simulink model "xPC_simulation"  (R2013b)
settings: Solver=FixedStepDiscrete  SolverMode=MultiTasking  StartTime=0.0  StopTime=inf  FixedStep=1/Param.Fs  RelTol=1e-3
InitFcn:
  | clear all; clc; close all;
  | Param  = Config_parameter();
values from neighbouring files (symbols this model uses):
  FFTLen = 2^(ceil(log(nFrmLen)/log(2)))    [DFT_FilterBank_Analysis_func.m]    (also in DFT_FilterBank_Synthesis_func.m; main_run3.m)
  nHopSize = size(in_frame_seg,1)    [DFT_FilterBank_Analysis_func.m]    (also in DFT_FilterBank_Synthesis_func.m = size(ref_out,1); main_run3.m = 16)
  nNumChs = size(ref_out,1)    [DFT_FilterBank_Analysis_func.m]    (also in DFT_FilterBank_Synthesis_func.m = size(in_frame,2); main_run3.m = 32; OLA_func.m = size(in_frame,2); PDbranchingsmooth_sm.m = size(x,1))
undefined symbols (not defined in the file or in its folder): a_dd, AFC_switch, DownSample_factor, DownSamplingFactor, eta, Freq_shift, Fs, Input, mu, prototype_win, Range, VarAmpSwitch, VarAttackTime, VarCompressRatio, VarCompressTh, VarFs, VarKneeWidth, VarLimiterCompressRatio, VarLimiterTh, VarMaxSPL, VarMicNoiseCompressRatio, VarMicNoiseTh, VarRefGaindB, VarRefSPL, VarReleaseTime, VarSwitch, VarThdB, Wiener_switch
libraries: xpcgeneralstandardslib x2, dspadpt3 x1, dspbuff3 x1, xpclib x1

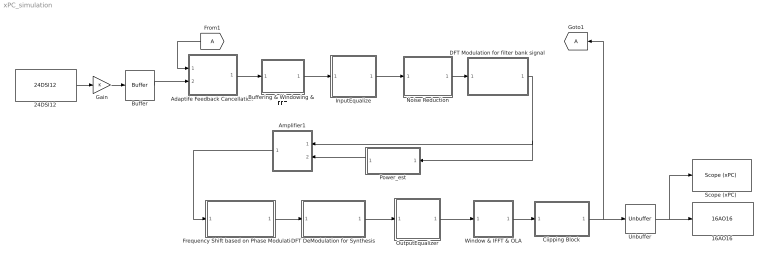
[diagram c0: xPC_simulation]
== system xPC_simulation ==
  "16AO16 " : xpcgeneralstandardslib/Audio/16AO16   channel=[1]  range=+-10.0  gsense=off  clksrc=External: slave to 24DSI12  framesize=1  samplerate=Param.Fs  sampletime=-1  autocal=on  extsync=LVDS  slot=-1
  24DSI12 : xpcgeneralstandardslib/Audio/24DSI12  channel=[1]  range=+-10.0  framesize=1  samplerate=Param.Fs  sampletime=-1  convert="+-Input Range (+-10  +-5 or +-2.5)"  filter=Low Frequency  mode=Hardware clock/Initiator  autocal=on  extsync=LVDS  slot=-1
  Adaptife Feedback Cancellation : Subsystem
  Amplifier1 : Subsystem
  Buffer : Buffer  N=Param.IO_FrameSize  TreatMby1Signals=One channel
  Buffering & Windowing &  FFT : Subsystem
  Ciipping Block : Subsystem
  DFT DeModulation for Synthesis : Subsystem
  DFT Modulation for filter bank signal : Subsystem
  Frequency Shift based on Phase Modulation : Subsystem
  From1 : From
  Gain : Gain
  Goto1 : Goto
  InputEqualize : MATLAB Function  TreatAsAtomicUnit=on
  Noise Reduction : Subsystem
  OutputEqualizer : MATLAB Function  TreatAsAtomicUnit=on
  Power_est : Subsystem
  "Scope (xPC) " : xpclib/Misc./Scope (xPC)   scopeno=1  scopetype=Target  autostart=on  viewmode=Graphical redraw  formatstr='%15.6f'  grid=on  ylimits=[0,0]  nosamples=250  noprepostsamples=0  interleave=1  triggermode=FreeRun  triggersignal=1  trigsignalfromport=off  triggerlevel=0.0  triggerslope=Either  triggerscope=1  triggersample=0  filename=data.dat  mode=Lazy  writesize=512  autorestart=off  dynamicfilemode=off  maxwritefilesize=512*1024^2
  Unbuffer : Unbuffer  SampleBasedProcessing=Same as frame based
  Window & IFFT & OLA : Subsystem
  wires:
  24DSI12/1 -> Gain/1
  Unbuffer/1 -> "Scope (xPC) "/1, "16AO16 "/1
  Window & IFFT & OLA/1(Out1) -> Ciipping Block/1(In1)
  DFT DeModulation for Synthesis/1(Out1) -> OutputEqualizer/1(InFreq)
  Frequency Shift based on Phase Modulation/1(Out1) -> DFT DeModulation for Synthesis/1(In1)
  DFT Modulation for filter bank signal/1(Out1) -> Amplifier1/1(In1), Power_est/1(In1)
  Amplifier1/1(Out1) -> Frequency Shift based on Phase Modulation/1(In1)
  Noise Reduction/1(Out1) -> DFT Modulation for filter bank signal/1(In1)
  Buffering & Windowing &  FFT/1(Out1) -> InputEqualize/1(InFreq)
  From1/1 -> Adaptife Feedback Cancellation/1(In1)
  Adaptife Feedback Cancellation/1(Out1) -> Buffering & Windowing &  FFT/1(In1)
  InputEqualize/1(OutFreqCal) -> Noise Reduction/1(In1)
  OutputEqualizer/1(OutFreqCal) -> Window & IFFT & OLA/1(In1)
  Ciipping Block/1(Out1) -> Unbuffer/1, Goto1/1
  Power_est/1(Out1) -> Amplifier1/2(In2)
  Buffer/1 -> Adaptife Feedback Cancellation/2(In2)
  Gain/1 -> Buffer/1

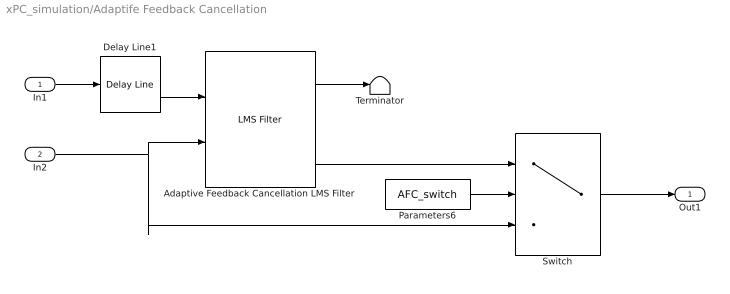
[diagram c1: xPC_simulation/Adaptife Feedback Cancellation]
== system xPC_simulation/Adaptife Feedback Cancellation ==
  In1 : Inport
  In2 : Inport  Port=2
  Adaptive Feedback Cancellation LMS Filter : dspadpt3/LMS Filter  Algo=LMS  L=Param.nFrmLen  stepflag=Dialog  mu=0.002  leakage=1.0  ic=0  Adapt=off  resetflag=None  weights=off  secondCoeffMode=User-defined  secondCoeffWordLength=2  secondCoeffFracLength=15  accum2Mode=User-defined  accum2FracLength=20  prodOutput2Mode=User-defined  prodOutput2FracLength=20  prodOutput3Mode=User-defined  prodOutput3FracLength=20  prodOutput4Mode=User-defined  prodOutput4FracLength=20  quotientMode=User-defined  quotientFracLength=20  roundingMode=Floor  overflowMode=off  addnparflag=off
  Delay Line1 : dspbuff3/Delay Line  siz=Param.IO_FrameSize  ic=0  directfeed=off  enable_output=off  hold_output=off  TreatMby1Signals=One channel
  Parameters6 : Constant  Value=AFC_switch
  Switch : Switch  Criteria=u2 > Threshold
  Terminator : Terminator
  Out1 : Outport
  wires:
  Parameters6/1 -> Switch/2
  Switch/1 -> Out1/1
  Delay Line1/1 -> Adaptive Feedback Cancellation LMS Filter/1
  Adaptive Feedback Cancellation LMS Filter/1 -> Terminator/1
  Adaptive Feedback Cancellation LMS Filter/2 -> Switch/1
  In1/1 -> Delay Line1/1
  In2/1 -> Switch/3, Adaptive Feedback Cancellation LMS Filter/2

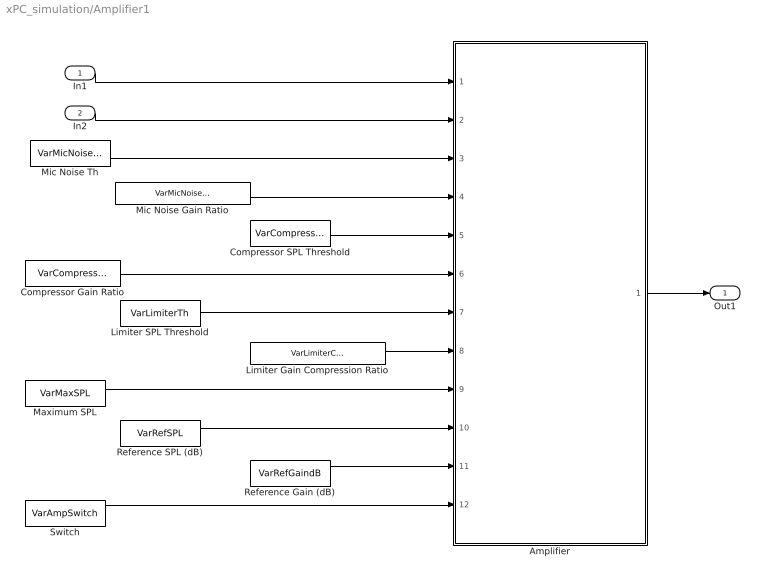
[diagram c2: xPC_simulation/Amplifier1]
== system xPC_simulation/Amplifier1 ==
  In1 : Inport
  In2 : Inport  Port=2
  Amplifier : MATLAB Function  TreatAsAtomicUnit=on
  Compressor Gain Ratio : Constant  Value=VarCompressRatio  VectorParams1D=off
  Compressor SPL Threshold : Constant  Value=VarCompressTh  VectorParams1D=off
  Limiter Gain Compression Ratio : Constant  Value=VarLimiterCompressRatio  VectorParams1D=off
  Limiter SPL Threshold : Constant  Value=VarLimiterTh  VectorParams1D=off
  Maximum SPL : Constant  Value=VarMaxSPL  VectorParams1D=off
  Mic Noise Gain Ratio : Constant  Value=VarMicNoiseCompressRatio  VectorParams1D=off
  Mic Noise Th : Constant  Value=VarMicNoiseTh  VectorParams1D=off
  Reference Gain (dB) : Constant  Value=VarRefGaindB  VectorParams1D=off
  Reference SPL (dB) : Constant  Value=VarRefSPL  VectorParams1D=off
  Switch : Constant  Value=VarAmpSwitch  VectorParams1D=off
  Out1 : Outport
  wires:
  In1/1 -> Amplifier/1(in_FBSig)
  Amplifier/1(Out_FBSig) -> Out1/1
  In2/1 -> Amplifier/2(in_EstdB)
  Compressor SPL Threshold/1 -> Amplifier/5(CT)
  Mic Noise Gain Ratio/1 -> Amplifier/4(ER)
  Mic Noise Th/1 -> Amplifier/3(ET)
  Reference Gain (dB)/1 -> Amplifier/11(G0)
  Reference SPL (dB)/1 -> Amplifier/10(L0)
  Maximum SPL/1 -> Amplifier/9(Lmax)
  Limiter Gain Compression Ratio/1 -> Amplifier/8(LR)
  Limiter SPL Threshold/1 -> Amplifier/7(LT)
  Compressor Gain Ratio/1 -> Amplifier/6(CR)
  Switch/1 -> Amplifier/12(AmpSwitch)

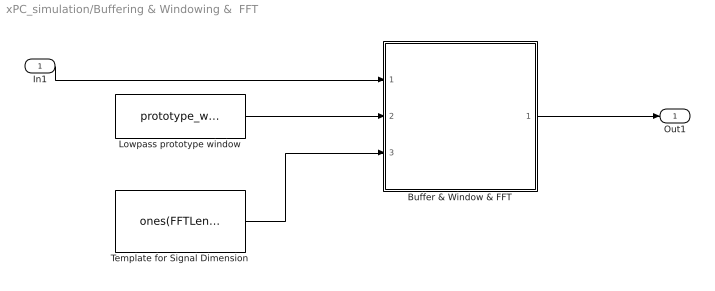
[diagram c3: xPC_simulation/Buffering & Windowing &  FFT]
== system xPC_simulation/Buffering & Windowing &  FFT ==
  In1 : Inport
  Buffer & Window & FFT : MATLAB Function  TreatAsAtomicUnit=on
  Lowpass prototype window : Constant  Value=prototype_win  VectorParams1D=off
  Template for Signal Dimension : Constant  Value=ones(FFTLen,nNumChs)  VectorParams1D=off
  Out1 : Outport
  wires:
  In1/1 -> Buffer & Window & FFT/1(in_frame_seg)
  Buffer & Window & FFT/1(FreqOut) -> Out1/1
  Template for Signal Dimension/1 -> Buffer & Window & FFT/3(ref_out)
  Lowpass prototype window/1 -> Buffer & Window & FFT/2(win)

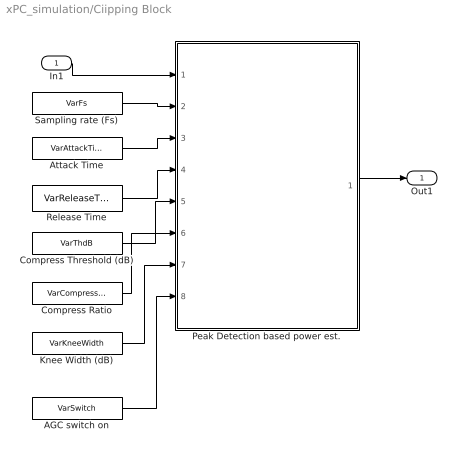
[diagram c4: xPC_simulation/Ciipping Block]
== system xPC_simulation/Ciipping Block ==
  In1 : Inport
  AGC switch on : Constant  Value=VarSwitch  VectorParams1D=off
  Attack Time : Constant  Value=VarAttackTime  VectorParams1D=off
  Compress Ratio : Constant  Value=VarCompressRatio  VectorParams1D=off
  Compress Threshold (dB) : Constant  Value=VarThdB  VectorParams1D=off
  Knee Width (dB) : Constant  Value=VarKneeWidth  VectorParams1D=off
  Peak Detection based power est. : MATLAB Function  TreatAsAtomicUnit=on
  Release Time : Constant  Value=VarReleaseTime  VectorParams1D=off
  Sampling rate (Fs) : Constant  Value=VarFs  VectorParams1D=off
  Out1 : Outport
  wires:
  In1/1 -> Peak Detection based power est./1(x)
  Peak Detection based power est./1(y) -> Out1/1
  Sampling rate (Fs)/1 -> Peak Detection based power est./2(fs)
  Attack Time/1 -> Peak Detection based power est./3(tauAttack)
  Release Time/1 -> Peak Detection based power est./4(tauRelease)
  Compress Threshold (dB)/1 -> Peak Detection based power est./5(Threshold)
  Knee Width (dB)/1 -> Peak Detection based power est./7(KneeWidth)
  Compress Ratio/1 -> Peak Detection based power est./6(ratio)
  AGC switch on/1 -> Peak Detection based power est./8(AGCSwitch)

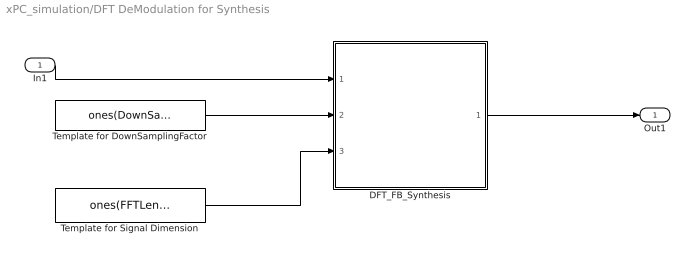
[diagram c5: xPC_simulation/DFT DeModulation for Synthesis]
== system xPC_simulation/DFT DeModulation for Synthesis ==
  In1 : Inport
  DFT_FB_Synthesis : MATLAB Function  TreatAsAtomicUnit=on
  Template for DownSamplingFactor : Constant  Value=ones(DownSample_factor,1)  VectorParams1D=off
  Template for Signal Dimension : Constant  Value=ones(FFTLen,nHopSize)  VectorParams1D=off
  Out1 : Outport
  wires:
  In1/1 -> DFT_FB_Synthesis/1(FB_In)
  DFT_FB_Synthesis/1(Out_FFTSig) -> Out1/1
  Template for DownSamplingFactor/1 -> DFT_FB_Synthesis/2(ref_DownSample_factor)
  Template for Signal Dimension/1 -> DFT_FB_Synthesis/3(ref_out)

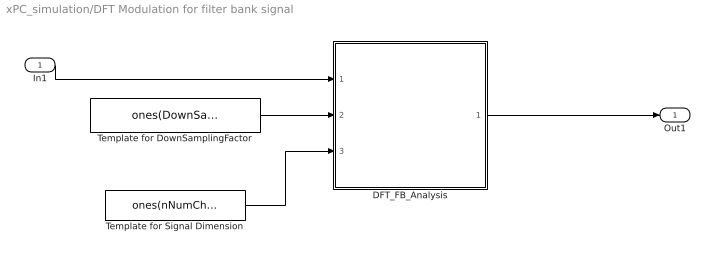
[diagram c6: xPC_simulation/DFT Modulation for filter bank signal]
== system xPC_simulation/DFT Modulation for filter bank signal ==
  In1 : Inport
  DFT_FB_Analysis : MATLAB Function  TreatAsAtomicUnit=on
  Template for DownSamplingFactor : Constant  Value=ones(DownSample_factor,1)  VectorParams1D=off
  Template for Signal Dimension : Constant  Value=ones(nNumChs,nHopSize)  VectorParams1D=off
  Out1 : Outport
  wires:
  Template for DownSamplingFactor/1 -> DFT_FB_Analysis/2(ref_DownSample_factor)
  Template for Signal Dimension/1 -> DFT_FB_Analysis/3(ref_out)
  DFT_FB_Analysis/1(FB_Out) -> Out1/1
  In1/1 -> DFT_FB_Analysis/1(in_FFTSig)

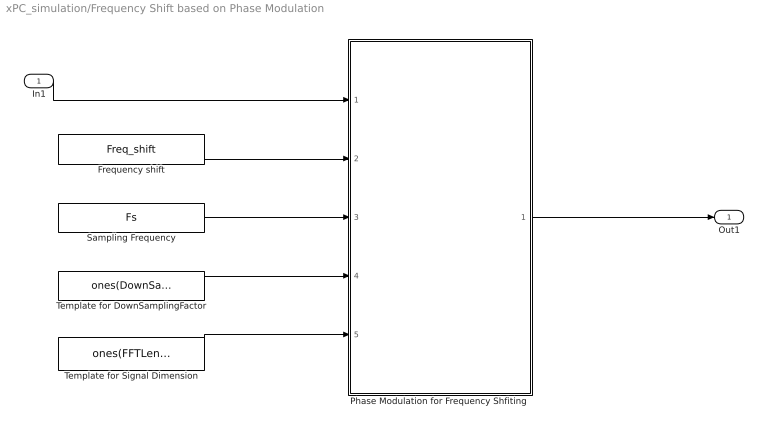
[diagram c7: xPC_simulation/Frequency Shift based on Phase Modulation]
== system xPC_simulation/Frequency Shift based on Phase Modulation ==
  In1 : Inport
  Frequency shift : Constant  Value=Freq_shift  VectorParams1D=off
  "Phase Modulation for Frequency Shfiting " : MATLAB Function  TreatAsAtomicUnit=on
  Sampling Frequency : Constant  Value=Fs  VectorParams1D=off
  Template for DownSamplingFactor : Constant  Value=ones(DownSample_factor,1)  VectorParams1D=off
  Template for Signal Dimension : Constant  Value=ones(FFTLen,nHopSize)  VectorParams1D=off
  Out1 : Outport
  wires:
  In1/1 -> "Phase Modulation for Frequency Shfiting "/1(FB_In)
  "Phase Modulation for Frequency Shfiting "/1(FreqShiftOut) -> Out1/1
  Template for DownSamplingFactor/1 -> "Phase Modulation for Frequency Shfiting "/4(ref_Downsample_factor)
  Template for Signal Dimension/1 -> "Phase Modulation for Frequency Shfiting "/5(ref_out)
  Frequency shift/1 -> "Phase Modulation for Frequency Shfiting "/2(Pm_freq)
  Sampling Frequency/1 -> "Phase Modulation for Frequency Shfiting "/3(Fs)

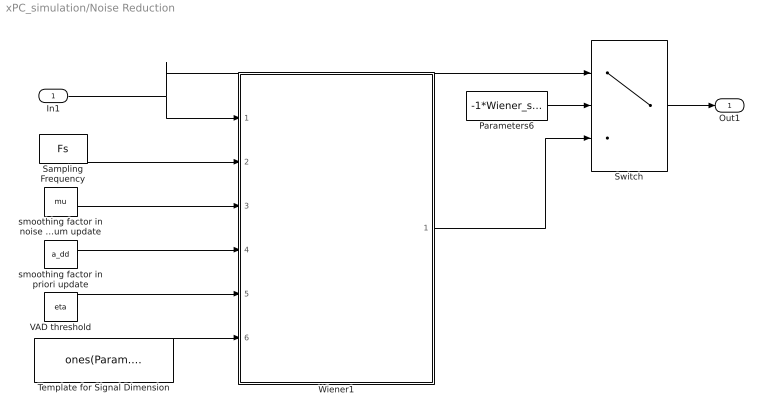
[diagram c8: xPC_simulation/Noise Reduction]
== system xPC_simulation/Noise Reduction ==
  In1 : Inport
  Parameters6 : Constant  Value=-1*Wiener_switch
  Sampling Frequency : Constant  Value=Fs  VectorParams1D=off
  Switch : Switch
  Template for Signal Dimension : Constant  Value=ones(Param.IO_FrameSize,1)  VectorParams1D=off
  VAD threshold : Constant  Value=eta  VectorParams1D=off
  Wiener1 : MATLAB Function  TreatAsAtomicUnit=on
  smoothing factor in noise spectrum update : Constant  Value=mu  VectorParams1D=off
  smoothing factor in priori update : Constant  Value=a_dd  VectorParams1D=off
  Out1 : Outport
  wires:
  In1/1 -> Switch/1, Wiener1/1(NoisyFreq)
  Sampling Frequency/1 -> Wiener1/2(Fs)
  Wiener1/1(EnhanFreq) -> Switch/3
  smoothing factor in noise spectrum update/1 -> Wiener1/3(mu)
  smoothing factor in priori update/1 -> Wiener1/4(a_dd)
  VAD threshold/1 -> Wiener1/5(eta)
  Template for Signal Dimension/1 -> Wiener1/6(ref_out)
  Switch/1 -> Out1/1
  Parameters6/1 -> Switch/2

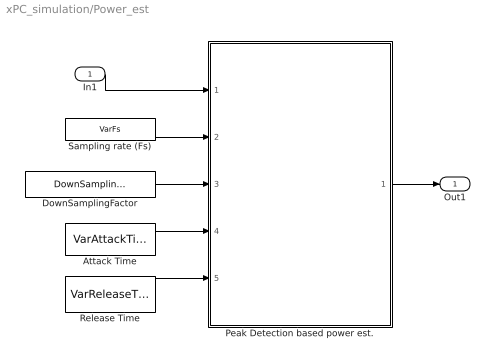
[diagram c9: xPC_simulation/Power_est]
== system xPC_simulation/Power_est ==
  In1 : Inport
  Attack Time : Constant  Value=VarAttackTime  VectorParams1D=off
  DownSamplingFactor : Constant  Value=DownSamplingFactor  VectorParams1D=off
  Peak Detection based power est. : MATLAB Function  TreatAsAtomicUnit=on
  Release Time : Constant  Value=VarReleaseTime  VectorParams1D=off
  Sampling rate (Fs) : Constant  Value=VarFs  VectorParams1D=off
  Out1 : Outport
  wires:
  In1/1 -> Peak Detection based power est./1(x)
  Peak Detection based power est./1(lg) -> Out1/1
  Sampling rate (Fs)/1 -> Peak Detection based power est./2(fs)
  Attack Time/1 -> Peak Detection based power est./4(tauAttack)
  Release Time/1 -> Peak Detection based power est./5(tauRelease)
  DownSamplingFactor/1 -> Peak Detection based power est./3(DownSamplingFactor)

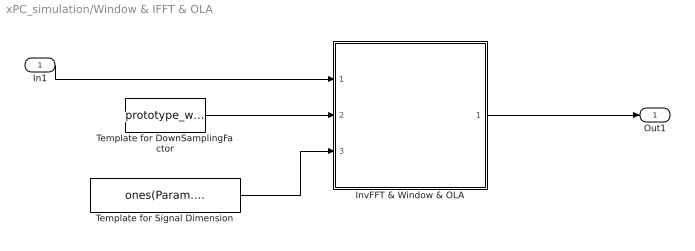
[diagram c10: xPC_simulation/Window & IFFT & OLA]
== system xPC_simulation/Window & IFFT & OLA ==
  In1 : Inport
  InvFFT & Window & OLA : MATLAB Function  TreatAsAtomicUnit=on
  Template for DownSamplingFactor : Constant  Value=prototype_win  VectorParams1D=off
  Template for Signal Dimension : Constant  Value=ones(Param.IO_FrameSize,1)  VectorParams1D=off
  Out1 : Outport
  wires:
  Template for Signal Dimension/1 -> InvFFT & Window & OLA/3(ref_out)
  Template for DownSamplingFactor/1 -> InvFFT & Window & OLA/2(win)
  InvFFT & Window & OLA/1(TimeSegOut) -> Out1/1
  In1/1 -> InvFFT & Window & OLA/1(FreqIn)
